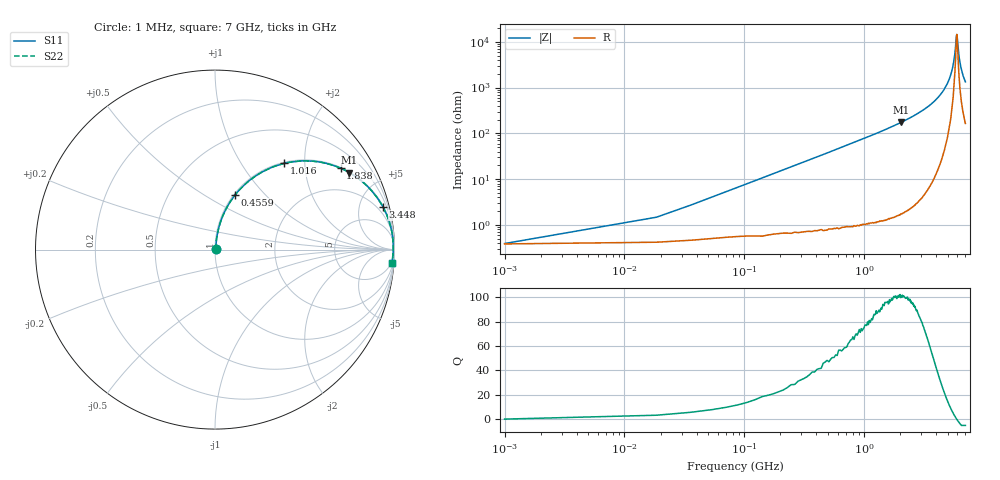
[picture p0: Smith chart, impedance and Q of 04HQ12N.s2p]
! Coilcraft 0403HQ-12N Chip Inductor
! 13 February 2004
# MHZ S MA R 50
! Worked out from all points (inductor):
!   401 points, 1 MHz to 7 GHz, reference 50 ohm
!   read as one part in series: L = 11.9 nH near 35.99 MHz
!   highest Q = 101 at 2.031 GHz (marker M1), where L = 13.6 nH
!   self-resonance near 5.933 GHz
!   S11 on the Smith chart (normalised r, x): 1 MHz: 1.01, +0.00; 455.9 MHz: 1.02, +0.69; 1.016 GHz: 1.02, +1.58; 1.838 GHz: 1.03, +3.07; 3.448 GHz: 1.14, +7.85; 7 GHz: 4, -27
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1  0.003761 11.5  0.996 -0.0  0.996 -0.0  0.003761 11.5
53.492  0.04 80.7  0.994 -2.3  0.994 -2.3  0.04 80.7
88.487  0.066 81.6  0.992 -3.8  0.992 -3.8  0.066 81.6
123.482  0.092 81.2  0.99 -5.3  0.99 -5.3  0.092 81.2
263.462  0.194 76.9  0.974 -11.2  0.974 -11.2  0.194 76.9
455.935  0.325 69.8  0.939 -18.9  0.939 -18.9  0.325 69.8
1015.855  0.616 51.3  0.78 -38.0  0.78 -38.0  0.616 51.3
1173.332  0.673 47.0  0.731 -42.3  0.731 -42.3  0.673 47.0
1838.237  0.834 32.9  0.544 -56.5  0.544 -56.5  0.834 32.9
2030.71  0.863 29.8  0.497 -59.6  0.497 -59.6  0.863 29.8
2345.665  0.899 25.4  0.429 -64.0  0.429 -64.0  0.899 25.4
3448.007  0.965 14.2  0.246 -74.9  0.246 -74.9  0.965 14.2
3500.5  0.967 13.8  0.239 -75.2  0.239 -75.2  0.967 13.8
4672.833  0.989 6.1  0.107 -81.2  0.107 -81.2  0.989 6.1
5407.728  0.993 2.4  0.042 -79.4  0.042 -79.4  0.993 2.4
5670.19  0.993 1.2  0.021 -71.2  0.021 -71.2  0.993 1.2
5845.165  0.993 0.4  0.009466 -44.3  0.009466 -44.3  0.993 0.4
5950.15  0.993 -0.1  0.007029 10.1  0.007029 10.1  0.993 -0.1
6177.618  0.992 -1.0  0.019 66.6  0.019 66.6  0.992 -1.0
6352.593  0.992 -1.7  0.031 74.0  0.031 74.0  0.992 -1.7
6615.055  0.991 -2.8  0.049 77.5  0.049 77.5  0.991 -2.8
7000  0.988 -4.2  0.074 78.7  0.074 78.7  0.988 -4.2
